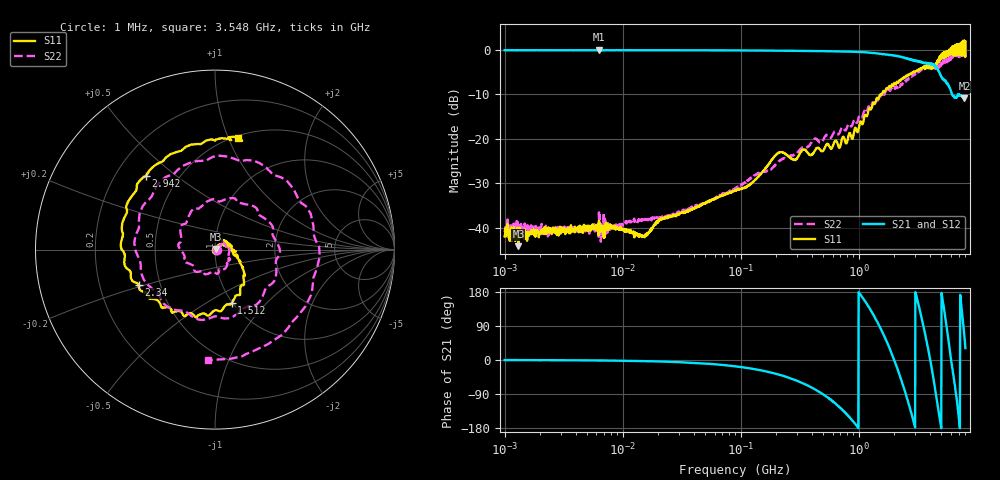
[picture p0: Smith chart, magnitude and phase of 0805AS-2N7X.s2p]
!s-Parameter Generated by FASTRON Sdn. Bhd.
!FASTRON P/N : 0805AS-2N7X
!Keysight Technologies: E5071C_MY46733604_B.14.02
!Date: Mon Jun 15 12:46:12 2026
!Version  :Rev01  Mon Jun 15 12:46:12 2026
!Data & Calibration Information:
!Freq  S11:SOLT2(ON)  S21:SOLT2(ON)  S12:SOLT2(ON)  S22:SOLT2(ON)
!PortZ  Port1:50+j0  Port2:50+j0
!When reading reference impedance value at option line is always used.
! Remarks : This data is being provided solely for informational purposes.
# Hz S dB R 50
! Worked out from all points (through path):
!   1601 points, 1 MHz to 8 GHz, reference 50 ohm
!   highest |S21| = 0.06 dB at 6.301 MHz (marker M1); lowest = -10.9 dB at 7.846 GHz (marker M2)
!   group delay of S21, straight-line fit = 493 ps
!   lowest |S11| = -44.1 dB at 1.31 MHz (marker M3), VSWR 1.01, Z = 50.6 + j0.287 ohm
!   |S11| at or under -10 dB: start of sweep to 1.518 GHz; 1.543 GHz to 1.574 GHz (30.94 MHz wide, 1.99 % of centre)
!   |S22| runs from -43.1 to -0.5 dB; largest |S21 - S12| = 0.02
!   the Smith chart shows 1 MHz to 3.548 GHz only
!   S11 on the Smith chart (normalised r, x): 1 MHz: 1.02, +0.00; 1.512 GHz: 0.99, -0.65; 2.34 GHz: 0.38, -0.19; 2.942 GHz: 0.33, +0.40; 3.548 GHz: 0.52, +1.08
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1000000  -41.90 0.1  -0.09 -0.3  -0.08 -0.3  -40.90 -0.6
1310238  -44.10 27.1  -0.12 -0.0  -0.08 -0.3  -38.90 -10.3
4479405  -40.40 5.1  -0.09 -0.9  -0.09 -1.0  -40.50 7.8
6301378  -38.40 10.4  0.06 -1.2  -0.10 -1.6  -36.50 21.3
2.00676e7  -38.30 22.0  -0.10 -3.8  -0.11 -3.8  -37.90 27.7
8.994653e7  -31.50 49.1  -0.13 -16.7  -0.14 -16.7  -31.10 34.4
4.006501e8  -23.50 53.7  -0.27 -72.9  -0.27 -73.0  -20.70 -35.6
9.68578e8  -18.40 -12.6  -0.46 -175.0  -0.46 -175.0  -16.40 -145.0
1.511962e9  -10.10 -72.8  -0.91 86.6  -0.92 86.4  -10.30 68.3
1.7949e9  -8.31 -105.0  -1.19 36.0  -1.18 35.8  -8.81 -2.3
2.340174e9  -6.56 -155.0  -1.65 -62.1  -1.67 -62.2  -7.75 -147.0
2.941737e9  -4.97 133.0  -2.48 -168.0  -2.50 -168.0  -5.37 67.2
3.548043e9  -3.95 78.6  -3.02 85.6  -3.01 85.6  -4.19 -93.6
4.26866e9  -3.75 -10.2  -3.17 -45.4  -3.20 -45.9  -3.99 99.7
4.660546e9  -2.30 -44.1  -4.34 -121.0  -4.35 -121.0  -3.94 -15.2
5.136407e9  -1.06 -83.4  -6.46 159.0  -6.50 158.0  -2.81 -146.0
5.668252e9  -0.87 -149.0  -7.73 65.6  -7.74 65.3  -2.19 103.0
6.226476e9  0.81 175.0  -10.30 -23.9  -10.30 -24.9  -0.95 -55.8
6.804799e9  0.26 116.0  -10.40 -112.0  -10.50 -112.0  -1.12 -173.0
7.228903e9  1.15 79.2  -10.20 172.0  -10.20 173.0  -0.69 89.0
7.845781e9  -1.13 23.3  -10.90 61.2  -10.70 61.4  -1.12 -68.6
8e9  1.91 -3.6  -10.60 31.4  -10.50 31.1  -0.83 -118.0
